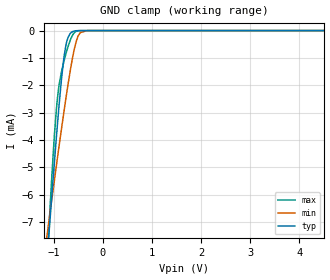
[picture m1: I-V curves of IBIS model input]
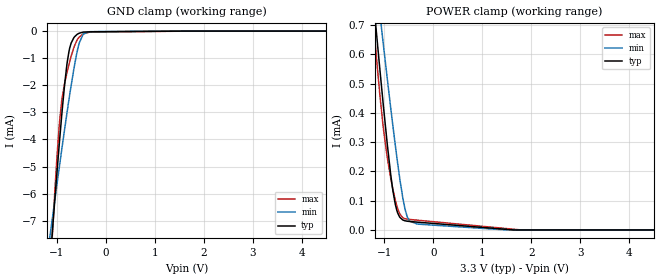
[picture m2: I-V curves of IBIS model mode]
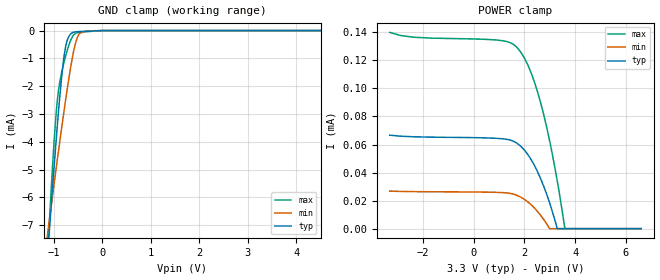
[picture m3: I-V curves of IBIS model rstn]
|Texas Instruments Incorporated
| 216kHz Digital Audio Interface Transceiver (DIX) with Stereo ADC and Routing
| Marketing part#   Digital Voltage Range   Package-type   #pins
| PCM9211PT   3.0V-3.6V   LQFP   48
| PCM9211PTR   3.0V-3.6V   LQFP   48
[IBIS Ver]   4.1
[File name]   pcm9211.ibs
[File Rev]   1.0
[Date]   9/19/2013
[Source]
| Texas Instruments Incorporated.
| Analog-eLab Design Center, HPA
| 12500 TI Blvd
| Dallas, TX -75243
[Notes]   Revision History:
| Rev 1.0: 9/19/2013
| - Initial version of the model
| - Model generated from simulations in SPECTRE
| - Model matched to SPECTRE simulation
| - C_comp although listed in numerical order of value are
|   obtained from varying PVT conditions. For PVT conditions for
|   each specific value refer the buffer description under
|   respective [Model]. IBIS model user is responsible for using
|   appropriate C_comp to simulate for Signal Integrity.
|*  EXCEPTION:   *
|*  - For model mode, there will be a leakage current in the GROUND   *
|*   clamp I-V Table because of mosfet M1 connected between PAD and   *
|*   Ground and there will be a leakage current in the POWER clamp   *
|*   I-V Table because of the mosfet M0 connected between PAD and VDD  *
|*  - For model rstn, there will be a leakage current in the POWER   *
|*   clamp I-V Table because of the mosfet MNPUDN connected between   *
|*   PAD and Ground   *
[Disclaimer]
| This model is designed as an aid for customers of Texas Instruments.
| TI and its licensors and suppliers make no warranties, either expressed
| or implied, with respect to this  model, including the warranties of
| merchantability or fitness for a particular purpose. The model is
| provided solely on an "as is" basis. The entire risk as to its quality
| and performance is with the customer.
[Copyright]
(C) Copyright 2013 Texas Instruments Incorporated.All rights reserved.
|   PCM9211PT
[Component]   PCM9211PT
[Manufacturer]   TI
[Package]   |48 LQFP  -  PT package
|   typ   min   max
R_pkg   0.13502   0.12243   0.17221
L_pkg   3.32278nH   2.89818nH   4.48397nH
C_pkg   0.51500pF   0.42914pF   0.62866pF
[Pin]  signal_name   model_name   R_pin   L_pin   C_pin
1   ERROR/INT0   tristate   0.17221   4.48397nH  0.62866pF
2   NPCM/INT1   tristate   0.15567   3.68220nH  0.56306pF
3   MPIO_A0   inout   0.14506   3.45256nH  0.53641pF
4   MPIO_A1   inout   0.13718   3.31964nH  0.52389pF
5   MPIO_A2   inout   0.13089   3.04548nH  0.47217pF
6   MPIO_A3   inout   0.12763   2.96290nH  0.42914pF
7   MPIO_C0   inout   0.12812   2.97028nH  0.42980pF
8   MPIO_C1   inout   0.12457   2.93380nH  0.46500pF
9   MPIO_C2   inout   0.12403   3.09003nH  0.50711pF
10   MPIO_C3   inout   0.12546   3.10823nH  0.51223pF
11   MPIO_B0   inout   0.13033   3.23380nH  0.53551pF
12   MPIO_B1   inout   0.14157   3.93531nH  0.60583pF
13   MPIO_B2   inout   0.14939   4.08845nH  0.60420pF
14   MPIO_B3   inout   0.13628   3.34721nH  0.53691pF
15   MPO0   tristate   0.12949   3.18610nH  0.51489pF
16   MPO1   tristate   0.12594   3.12749nH  0.51158pF
17   DOUT   tristate   0.12447   2.93908nH  0.46514pF
18   LRCK   tristate   0.12609   2.94208nH  0.43420pF
19   BCK   tristate   0.12889   2.98994nH  0.43748pF
20   SCKO   tristate   0.13297   3.08769nH  0.46631pF
21   DGND   gnd   0.06629   2.72112nH  0.55607pF
22   DVDD   power   0.04672   2.67934nH  0.60063pF
23   MDO/ADR0   inout   0.13033   3.23880nH  0.53686pF
24   MDI/SDA   inout   0.14160   3.94142nH  0.60209pF
25   MC/SCL   input   0.15050   4.10407nH  0.60908pF
26   MS/ADR1   input   0.13607   3.34020nH  0.54152pF
27   MODE   mode   0.12828   3.16036nH  0.51818pF
28   RXIN7/ADIN0   input   0.12414   3.09284nH  0.51055pF
29   RXIN6/ALRCKI0   input   0.12243   2.89818nH  0.46514pF
30   RXIN5/ABCKI0   input   0.12429   2.90460nH  0.43512pF
31   RXIN4/ASCKI0   input   0.12772   2.96288nH  0.43977pF
32   RXIN3   input   0.13276   3.07660nH  0.47853pF
33   RXIN2   input   0.14104   3.38733nH  0.53073pF
34   _RST   rstn   0.15094   3.55503nH  0.53384pF
35   RXIN1   input   0.14057   3.41000nH  0.53085pF
36   VDDRX   power   0.14592   4.00631nH  0.60671pF
37   RXIN0   input   0.14362   3.97582nH  0.59827pF
38   GNDRX   gnd   0.12557   3.14846nH  0.52041pF
39   XTI   nc   0.12258   3.05433nH  0.50664pF
40   XTO   nc   0.12168   3.04319nH  0.50954pF
41   AGND   gnd   0.06440   2.50716nH  0.52152pF
42   VCC   power   0.06555   2.43404nH  0.49818pF
43   FILT   nc   0.06570   2.52816nH  0.47619pF
44   VCOM   nc   0.12604   2.95559nH  0.46929pF
45   AGNDAD   gnd   0.04751   2.72902nH  0.60765pF
46   VCCAD   power   0.04761   2.65034nH  0.61264pF
47   VINL   nc   0.12978   3.21897nH  0.53374pF
48   VINR   nc   0.14235   3.94434nH  0.60392pF
| Models and submodels in the file (5): input (Input), mode (Input), rstn (Input), tristate (3-state), inout (I/O)
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|   input Model
[Model]   input
Model_type   Input
Vinl = 0.8
Vinh = 2.0
|   typ   min   max
|   (nom PVT)   (fast PVT)   (slow PVT)
C_comp   1.510e-13   3.511e-15   2.399e-13
| Where nom  PVT is Nominal Process, 3.3V, 27C
|   Fast PVT is Strong Process,  3.6V, -40C
|   Slow PVT is Weak Process,   3V, 150C
[Voltage Range]   3.3   3   3.6
|Junction Temperature
[Temperature Range]   27   150   -40
[Power Clamp Reference]   3.3   3   3.6
[GND Clamp Reference]   0   0   0
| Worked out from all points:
|   GND clamp passes 1 mA (typ) near -0.80 V on its own axis
[GND Clamp]
|   Voltage   I(typ)   I(min)   I(max)
-3.3V     -60.28mA   -36.6mA    -82.36mA
-1.128V   -8.106mA   -7.336mA   -8.131mA
-1.101V   -7.461mA   -6.973mA   -7.232mA
-1.093V   -7.274mA   -6.869mA   -6.976mA
-986.7mV  -4.766mA   -5.444mA   -3.781mA
-902.4mV  -2.912mA   -4.338mA   -2.102mA
-834.9mV  -1.613mA   -3.474mA   -1.431mA
-752.4mV  -520.5uA   -2.457mA   -839.6uA
-607.2mV  -28.18uA   -886.7uA   -133.4uA
-504mV    -1.828uA   -195.2uA   -7.266uA
-330mV    0A         -2.455uA   0A
6.6V      0A         0A         0A
[POWER Clamp]
|   Voltage   I(typ)   I(min)   I(max)
-3.3V     0A         0A         0A
0V        0A         0A         0A
6.6V      0A         0A         0A
|   mode Model
[Model]   mode
Model_type   Input
Vinl = 0.8
Vinh = 2.0
|   typ   min   max
|   (nom PVT)   (fast PVT)   (slow PVT)
C_comp   1.455e-13   3.454e-15   2.331e-13
| Where nom  PVT is Nominal Process, 3.3V, 27C
|   Fast PVT is Strong Process,  3.6V, -40C
|   Slow PVT is Weak Process,   3V, 150C
[Voltage Range]   3.3   3   3.6
|Junction Temperature
[Temperature Range]   27   150   -40
[Power Clamp Reference]   3.3   3   3.6
[GND Clamp Reference]   0   0   0
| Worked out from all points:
|   GND clamp passes 1 mA (typ) near -0.78 V on its own axis
|   POWER clamp passes 1 mA (typ) near -1.34 V on its own axis
[GND Clamp]
|   Voltage   I(typ)   I(min)   I(max)
-3.3V     -60.32mA   -36.63mA   -82.44mA
-1.116V   -7.913mA   -7.199mA   -8.211mA
-1.054V   -6.443mA   -6.363mA   -6.209mA
-951mV    -4.115mA   -5mA       -3.413mA
-897.6mV  -2.99mA    -4.304mA   -2.494mA
-798.6mV  -1.25mA    -3.051mA   -1.552mA
-744mV    -655.6uA   -2.389mA   -1.149mA
-654mV    -237.2uA   -1.38mA    -599.1uA
-546mV    -78.16uA   -442.8uA   -222.7uA
-462mV    -37.32uA   -104.7uA   -102.8uA
-318mV    -26.73uA   -21.96uA   -34.69uA
6.6V      0A         0A         0A
[POWER Clamp]
|   Voltage   I(typ)   I(min)   I(max)
-3.3V     4.73mA     4.147mA    5.247mA
-1.272V   870.2uA    1.006mA    805.7uA
-1.176V   694.6uA    860.6uA    613.2uA
-1.092V   544.3uA    734.9uA    457.7uA
-1.033V   441.5uA    647.5uA    362.1uA
-841.2mV  149.3uA    373.1uA    149.4uA
-745.8mV  65.71uA    246.3uA    80.93uA
-620.4mV  33.69uA    104.5uA    41.41uA
-489mV    29.05uA    30.31uA    36.01uA
-318mV    26.6uA     20.1uA     33.25uA
1.798V    0A         0A         0A
6.6V      0A         0A         0A
|   rstn Model
[Model]   rstn
Model_type   Input
Vinl = 0.8
Vinh = 2.0
|   typ   min   max
|   (nom PVT)   (fast PVT)   (slow PVT)
C_comp   1.510e-13   3.511e-15   2.399e-13
| Where nom  PVT is Nominal Process, 3.3V, 27C
|   Fast PVT is Strong Process,  3.6V, -40C
|   Slow PVT is Weak Process,   3V, 150C
[Voltage Range]   3.3   3   3.6
|Junction Temperature
[Temperature Range]   27   150   -40
[Power Clamp Reference]   3.3   3   3.6
[GND Clamp Reference]   0   0   0
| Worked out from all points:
|   GND clamp passes 1 mA (typ) near -0.79 V on its own axis
[GND Clamp]
|   Voltage   I(typ)   I(min)   I(max)
-3.3V     -60.28mA   -36.6mA    -82.37mA
-1.151V   -8.656mA   -7.643mA   -8.922mA
-1.099V   -7.416mA   -6.947mA   -7.192mA
-993.3mV  -4.926mA   -5.534mA   -4.007mA
-952.8mV  -4.01mA    -4.998mA   -3.028mA
-906mV    -3mA       -4.387mA   -2.209mA
-838.2mV  -1.688mA   -3.518mA   -1.517mA
-755.7mV  -580.5uA   -2.5mA     -920.7uA
-607.2mV  -70.15uA   -893uA     -199.2uA
-507mV    -38.42uA   -218uA     -71.98uA
-330mV    -23.18uA   -13.16uA   -41.59uA
6.6V      0A         0A         0A
[POWER Clamp]
|   Voltage   I(typ)   I(min)   I(max)
-3.3V     66.69uA    26.77uA    140uA
-2.353V   65.52uA    26.42uA    136.5uA
858mV     64.48uA    25.91uA    134.6uA
1.647V    61.64uA    24.2uA     130.3uA
1.87V     58.61uA    22.38uA    125.7uA
2.122V    53.28uA    19.32uA    117.4uA
2.41V     44.64uA    14.48uA    103.9uA
2.633V    35.99uA    9.701uA    90.35uA
2.997V    18.22uA    0A         62.53uA
3.297V    0A         0A         33.93uA
3.598V    0A         0A         0A
6.6V      0A         0A         0A
